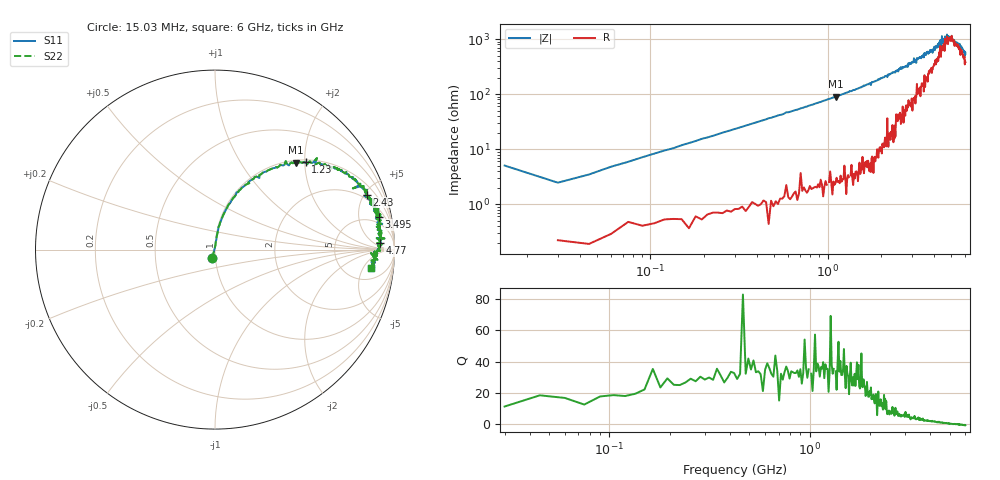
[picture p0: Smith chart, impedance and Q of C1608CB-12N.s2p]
!	Network	Analyzer	HP8753E.07.74:	Oct	30	2002	Serial	No.	JP38451487
!	Hewlett-Packard
!	7	Sep	2009	9:35:38
!	Frequency	S11	S21	S12	S22
#	HZ	S	RI	R	50
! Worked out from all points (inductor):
!   400 points, 15.03 MHz to 6 GHz, reference 50 ohm
!   read as one part in series: L = 12.5 nH near 45.03 MHz
!   highest Q = 36.4 at 1.11 GHz (marker M1), where L = 12.9 nH
!   self-resonance near 4.992 GHz
!   S11 on the Smith chart (normalised r, x): 15.03 MHz: 0.97, -0.09; 1.23 GHz: 1.06, +2.02; 2.43 GHz: 1.62, +5.22; 3.495 GHz: 3.21, +9.02; 4.77 GHz: 19, +9; 6 GHz: 9, -8
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1.502992e7  -0.0154 -0.0482  1.02 0.0482  1.02 0.0482  -0.0154 -0.0482
3.002985e7  0.00262 0.0244  0.997 -0.0244  0.997 -0.0244  0.00262 0.0244
7.502962e7  0.00832 0.0581  0.992 -0.0581  0.992 -0.0581  0.00832 0.0581
1.500292e8  0.0186 0.115  0.981 -0.115  0.981 -0.115  0.0186 0.115
3.600282e8  0.0789 0.254  0.921 -0.254  0.921 -0.254  0.0789 0.254
1.020025e9  0.402 0.475  0.598 -0.475  0.598 -0.475  0.402 0.475
1.110024e9  0.449 0.484  0.551 -0.484  0.551 -0.484  0.449 0.484
1.230024e9  0.505 0.486  0.495 -0.486  0.495 -0.486  0.505 0.486
2.01002e9  0.777 0.39  0.223 -0.39  0.223 -0.39  0.777 0.39
2.430018e9  0.846 0.306  0.154 -0.306  0.154 -0.306  0.846 0.306
3.015015e9  0.911 0.227  0.0894 -0.227  0.0894 -0.227  0.911 0.227
3.495013e9  0.915 0.182  0.0854 -0.182  0.0854 -0.182  0.915 0.182
4.00501e9  0.925 0.104  0.0755 -0.104  0.0755 -0.104  0.925 0.104
4.335008e9  0.921 0.055  0.0786 -0.055  0.0786 -0.055  0.921 0.055
4.365008e9  0.913 0.0869  0.0867 -0.0869  0.0867 -0.0869  0.913 0.0869
4.425008e9  0.944 0.0619  0.0562 -0.0619  0.0562 -0.0619  0.944 0.0619
4.455008e9  0.911 0.0659  0.0885 -0.0659  0.0885 -0.0659  0.911 0.0659
4.575007e9  0.901 0.0645  0.099 -0.0645  0.099 -0.0645  0.901 0.0645
4.605007e9  0.924 0.0327  0.0761 -0.0327  0.0761 -0.0327  0.924 0.0327
4.770006e9  0.917 0.0348  0.0827 -0.0348  0.0827 -0.0348  0.917 0.0348
5.010005e9  0.912 0.00388  0.0883 -0.00388  0.0883 -0.00388  0.912 0.00388
6e9  0.871 -0.101  0.129 0.101  0.129 0.101  0.871 -0.101
